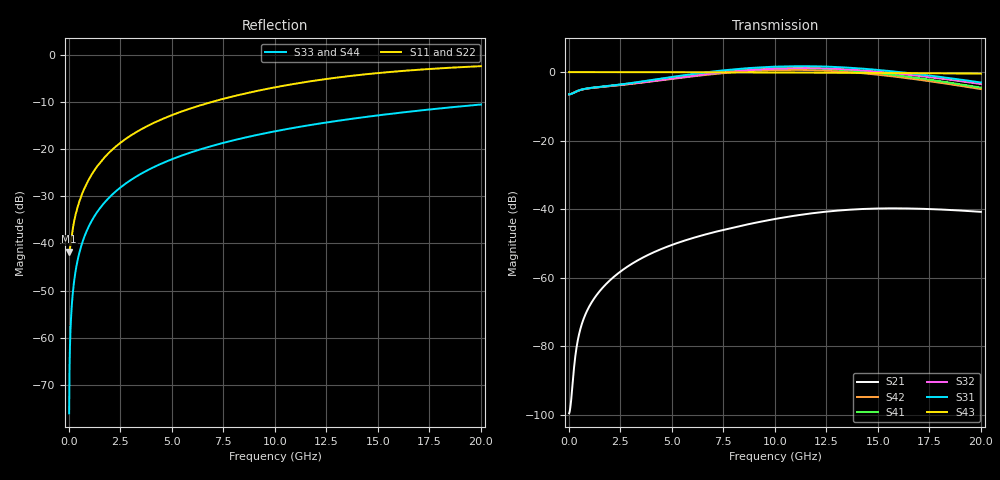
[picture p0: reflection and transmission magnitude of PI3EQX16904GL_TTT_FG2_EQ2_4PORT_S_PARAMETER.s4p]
! NPort=4 DATA=2000 NOISE=0 GROUPDELAY=0 COMPLEX_DATAFORMAT=POLAR
! NumOfBlock=1 NumOfParam=0
! .MODEL Smodel S TSTONEFILE=PI3EQX16904GL_TTT_FG2_EQ2_4PORT_S_PARAMETER.s4p TYPE=S
!  -- The above .MODEL line can be used for the S element in the netlist.
! The s parameter is extracted from the linear redriver, it is not bi-directional; only s(4,1)s(4,2) and s(3,1)s(3,2)
! should be the insertion loss
!Port definition:
!Port1 = input+
!Port2 = input-
!Port3 = output+
!Port4 = output-
# Hz S MA R  50
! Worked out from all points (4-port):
!   2000 points, 10 MHz to 20 GHz, reference 50 ohm
!   strongest paths, dB at 10 MHz, 5.01 GHz, 10.01 GHz, 15.01 GHz, 20 GHz:
!     S43: 0.0, 0.0, -0.1, -0.3, -0.4
!     S31: -6.5, -1.4, 1.6, 0.6, -3.0
!     S32: -6.5, -1.9, 1.0, 0.1, -3.5
!     S41: -6.5, -1.5, 1.2, -0.3, -4.5
!     S42: -6.5, -2.0, 0.6, -0.8, -5.0
!     S21: -99.6, -50.4, -42.9, -39.8, -40.8
!   lowest |S11| = -41.7 dB at 10 MHz (marker M1), VSWR 1.02, Z = 49.2 - j0.0603 ohm
!   |S11| at or under -10 dB: start of sweep to 6.906 GHz
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1e7  0.008182 -175.7  1.05e-05 7.6  0 0.0  0 0.0
     1.05e-05 7.6  0.008182 -175.7  0 0.0  0 0.0
     0.4743 0.2  0.4743 -179.8  0.0001571 -90.0  1 -0.0
     0.4743 -179.8  0.4743 0.2  1 -0.0  0.0001571 -90.0
2e8  0.01483 -130.6  3.383e-05 105.8  0 0.0  0 0.0
     3.383e-05 105.8  0.01483 -130.6  0 0.0  0 0.0
     0.494 4.3  0.4938 -175.9  0.003142 -90.2  1 -0.2
     0.494 -176.1  0.4938 3.7  1 -0.2  0.003142 -90.2
6.2e8  0.03268 -112.4  0.0002073 113.7  0 0.0  0 0.0
       0.0002073 113.7  0.03268 -112.4  0 0.0  0 0.0
       0.5562 3.9  0.5548 -176.6  0.009738 -90.6  0.9999 -0.6
       0.5561 -177.2  0.5547 2.2  0.9999 -0.6  0.009738 -90.6
2.97e9  0.1383 -101.6  0.001536 96.2  0 0.0  0 0.0
        0.001536 96.1  0.1384 -101.6  0 0.0  0 0.0
        0.6889 -11.4  0.6733 166.6  0.0466 -92.8  0.9988 -2.7
        0.6858 163.3  0.6703 -18.8  0.9988 -2.7  0.0466 -92.8
1.033e10  0.4686 -113.8  0.007539 42.7  0 0.0  0 0.0
          0.007473 43.0  0.4676 -113.9  0 0.0  0 0.0
          1.21 -101.6  1.133 78.4  0.16 -99.6  0.9861 -9.2
          1.148 60.5  1.075 -119.5  0.9861 -9.2  0.16 -99.6
1.448e10  0.6275 -123.9  0.01017 4.7  0 0.0  0 0.0
          0.01012 5.3  0.6257 -123.8  0 0.0  0 0.0
          1.109 -165.9  1.047 14.7  0.2213 -103.3  0.9732 -12.8
          1.006 -10.3  0.9498 170.3  0.9732 -12.8  0.2213 -103.3
2e10  0.7623 -135.6  0.009183 -37.4  0 0.0  0 0.0
      0.009139 -36.7  0.7611 -135.5  0 0.0  0 0.0
      0.7055 118.9  0.671 -60.3  0.2986 -108.1  0.9506 -17.4
      0.594 -93.0  0.565 87.8  0.9506 -17.4  0.2986 -108.1
